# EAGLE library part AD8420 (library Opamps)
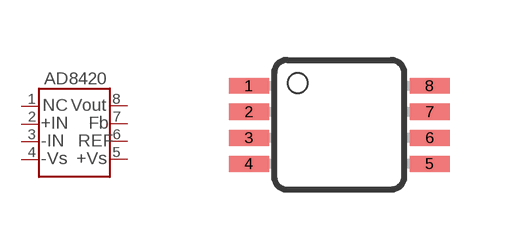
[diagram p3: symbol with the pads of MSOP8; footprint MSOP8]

Designator prefix U

## AD8420  [MSOP8]
1  1  nc
2  2  in
3  3  in
4  4  in
5  5  in
6  6  in
7  7  in
8  8  out

## Footprint MSOP8 (pad centres in mm)
smd 1 x 0.4: 1 -2.263,0.976; 2 -2.263,0.326; 3 -2.263,-0.324; 4 -2.263,-0.974; 5 2.262,-0.974; 6 2.262,-0.324; 7 2.262,0.326; 8 2.262,0.976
